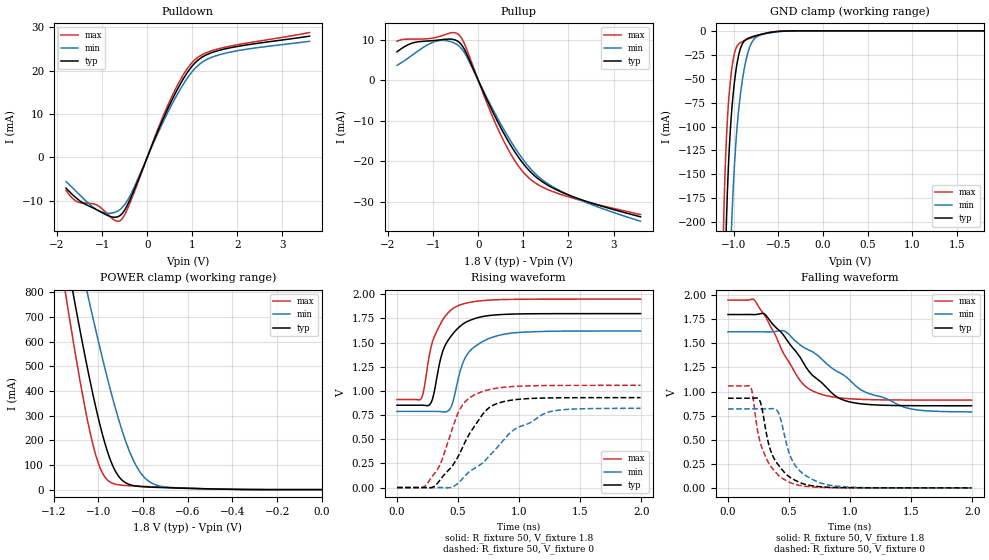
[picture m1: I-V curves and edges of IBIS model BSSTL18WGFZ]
[IBIS Ver] 3.2
[File Name] sprm450.ibs
[File Rev] 1.0
[Date] April 15, 2005
[Source] File Originated at Texas Instruments
[Disclaimer] Please be aware that in the absence of a written agreement
| Texas Instruments(TI) assumes no liability for:
| (1) The accuracy of the IBIS models provided to your company
| (2) The proper functioning of these Models in your design
| or for any resulting applications;or
| (3) Infringement of patents,copyrights, or intellectual
| property rights resulting from your use of these models.
| TI provides IBIS Models as a service to our customers and
| therefore reserves the right to limit distribution of the
| Models.
[Copyright] Property of Texas Instruments Incorporated.
| Unauthorized reproduction and/or distribution is strictly
| prohibited.
| This product is protected under copyright law and trade
| secret law as an unpublished work.
| Created 1999,(C) Copyright 1999-2000,
| Texas Instruments Incorporated., All Rights Reserved.
| These commodities are under the U.S.
| Government distribution license control.As such,they are not
| to be re-exported without the prior approval of the U.S.
| Department of Commerce.
[Notes] DDR Interface for DaVinci only
[Component] TL18WGFZ
[Manufacturer] Texas Instruments
[Package]
|Variable Typ Min Max
R_pkg 2.212e-01 1.101e-01 3.279e-01
L_pkg 4.011e-09 2.375e-09 5.798e-09
C_pkg 6.351e-13 3.910e-13 9.306e-13
[Pin] signal_name model_name
U1 DDR_D_BIT0 BSSTL18WGFZ
U2 DDR_D_BIT1 BSSTL18WGFZ
T5A VDDS1 POWER
W19A VSS GND
V1 DDR_D_BIT2 BSSTL18WGFZ
V2 DDR_D_BIT3 BSSTL18WGFZ
T4 DDR_DQM0 BSSTL18WGFZ
U4 DDR_DQS0 BSSTL18WGFZ
T5B VDDS1 POWER
W19B VSS GND
M12A VDD POWER
W2 DDR_D_BIT4 BSSTL18WGFZ
U3 DDR_D_BIT5 BSSTL18WGFZ
V3 DDR_D_BIT6 BSSTL18WGFZ
W3 DDR_D_BIT7 BSSTL18WGFZ
T5C VDDS1 POWER
W19C VSS GND
V4 DDR_D_BIT8 BSSTL18WGFZ
W4 DDR_D_BIT9 BSSTL18WGFZ
U5 DDR_D_BIT10 BSSTL18WGFZ
V5 DDR_D_BIT11 BSSTL18WGFZ
T5D VDDS1 POWER
W19D VSS GND
U6 DDR_DQS1 BSSTL18WGFZ
T6 DDR_DQM1 BSSTL18WGFZ
W5 DDR_D_BIT12 BSSTL18WGFZ
V6 DDR_D_BIT13 BSSTL18WGFZ
M12B VDD POWER
W19E VSS GND
T5E VDDS1 POWER
W6 DDR_D_BIT14 BSSTL18WGFZ
V7 DDR_D_BIT15 BSSTL18WGFZ
T7 DDR_CAS_N BSSTL18WGFZ
U7 DDR_RAS_N BSSTL18WGFZ
T8 DDR_WE_N BSSTL18WGFZ
W19F VSS GND
T5F VDDS1 POWER
T9 DDR_CS_N BSSTL18WGFZ
V8 DDR_CKE BSSTL18WGFZ
W19G VSS GND
W7 DDR_CLK0 BSSTL18WGFZ
W8 DDR_CLK0_N BSSTL18WGFZ
T5G VDDS1 POWER
W19H VSS GND
M12C VDD POWER
T10 DDR_VDDDLL NC
T11 DDR_VSSDLL NC
R8 DDR_AMUXDLL NC
U9 DDR_BS_BIT2 BSSTL18WGFZ
V9 DDR_BS_BIT1 BSSTL18WGFZ
U8 DDR_BS_BIT0 BSSTL18WGFZ
W19I VSS GND
T5H VDDS1 POWER
W9 DDR_A_BIT12 BSSTL18WGFZ
W10 DDR_A_BIT11 BSSTL18WGFZ
U10 DDR_A_BIT10 BSSTL18WGFZ
U11 DDR_A_BIT9 BSSTL18WGFZ
V10 DDR_A_BIT8 BSSTL18WGFZ
T12 DDR_PADREFN NC
T13 DDR_PADREFP NC
W19J VSS GND
T5I VDDS1 POWER
V11 DDR_A_BIT7 BSSTL18WGFZ
W11 DDR_A_BIT6 BSSTL18WGFZ
W12 DDR_A_BIT5 BSSTL18WGFZ
V12 DDR_A_BIT4 BSSTL18WGFZ
U12 DDR_A_BIT3 BSSTL18WGFZ
M12D VDD POWER
W19K VSS GND
T5J VDDS1 POWER
V13 DDR_A_BIT2 BSSTL18WGFZ
U13 DDR_A_BIT1 BSSTL18WGFZ
W13 DDR_A_BIT0 BSSTL18WGFZ
W14 DDR_D_BIT16 BSSTL18WGFZ
V14 DDR_D_BIT17 BSSTL18WGFZ
W19L VSS GND
T5K VDDS1 POWER
W15 DDR_D_BIT18 BSSTL18WGFZ
V15 DDR_D_BIT19 BSSTL18WGFZ
T14 DDR_DQM2 BSSTL18WGFZ
U14 DDR_DQS2 BSSTL18WGFZ
W19M VSS GND
T5L VDDS1 POWER
U15 DDR_D_BIT20 BSSTL18WGFZ
W16 DDR_D_BIT21 BSSTL18WGFZ
V16 DDR_D_BIT22 BSSTL18WGFZ
T17 DDR_D_BIT23 BSSTL18WGFZ
M12E VDD POWER
W19N VSS GND
T5M VDDS1 POWER
V17 DDR_D_BIT24 BSSTL18WGFZ
U17 DDR_D_BIT25 BSSTL18WGFZ
U18 DDR_D_BIT26 BSSTL18WGFZ
W17 DDR_D_BIT27 BSSTL18WGFZ
W19P VSS GND
T5N VDDS1 POWER
U16 DDR_DQS3 BSSTL18WGFZ
T16 DDR_DQM3 BSSTL18WGFZ
V18 DDR_D_BIT28 BSSTL18WGFZ
W18 DDR_D_BIT29 BSSTL18WGFZ
W19Q VSS GND
T15 VREFSSTL NC
T5P VDDS1 POWER
V19 DDR_D_BIT30 BSSTL18WGFZ
U19 DDR_D_BIT31 BSSTL18WGFZ
[Package Model] ddr
[Define Package Model] ddr
[Manufacturer] Texas Instruments Inc.
[OEM] Texas Instruments Inc.
[Description] Model for ddr generated by PACED 4.51F
[Number of Pins] 105
[Pin Numbers]
U1
U2
T5A
W19A
V1
V2
T4
U4
T5B
W19B
M12A
W2
U3
V3
W3
T5C
W19C
V4
W4
U5
V5
T5D
W19D
U6
T6
W5
V6
M12B
W19E
T5E
W6
V7
T7
U7
T8
W19F
T5F
T9
V8
W19G
W7
W8
T5G
W19H
M12C
T10
T11
R8
U9
V9
U8
W19I
T5H
W9
W10
U10
U11
V10
T12
T13
W19J
T5I
V11
W11
W12
V12
U12
M12D
W19K
T5J
V13
U13
W13
W14
V14
W19L
T5K
W15
V15
T14
U14
W19M
T5L
U15
W16
V16
T17
M12E
W19N
T5M
V17
U17
U18
W17
W19P
T5N
U16
T16
V18
W18
W19Q
T15
T5P
V19
U19
[Model Data]
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[End Model Data]
[End Package Model]
| Models and submodels in the file (1): BSSTL18WGFZ (I/O)
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|[Manufacturer] Texas Instruments.
|[Package]
| variable typ min max
|R_pkg 0.000 0.000 0.000
|L_pkg 0.000H 0.000H 0.000H
|C_pkg 0.000F 0.000F 0.000F
|[Pin] signal_name model_name R_pin L_pin C_pin
|PAD PAD BSSTL18WGFZ NA NA NA
|VDDS VDDS POWER NA NA NA
|VSSS VSSS GND NA NA NA
[Model] BSSTL18WGFZ
Model_type I/O
Polarity Non-Inverting
Enable Active-Low
Vinl = 0.6500V
Vinh = 1.1500V
Vmeas = 0.9000V
Cref = 5.0000pF
Rref = 50.0000
Vref = 0.9000V
| typ min max
|C_comp   1.0539pF   1.0159pF   1.1018pF
|  ADDED 80FF TO C_comp FOR DRIVER TO PAD CAP.
C_comp   1.1339pF   1.0959pF   1.1818pF
[Model Spec]
Vinh 1.1500V 1.0600V 1.2250V
Vinl 0.6500V 0.5600V 0.7250V
[Temperature Range] 25.0000 125.000 -40.0000
[Voltage Range] 1.8000V 1.6200V 1.9500V
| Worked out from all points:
|   slope of the pulldown table from 0 to 0.27 V, typ, clamps not added: 39.3 ohm
|   slope of the pullup table from 0 to 0.27 V, typ, clamps not added: 40.9 ohm
|   GND clamp passes 1 mA (typ) near -0.54 V on its own axis
|   POWER clamp passes 1 mA (typ) near -0.39 V on its own axis
|   rising waveform, R_fixture 50, V_fixture 1.8: 20-80 % time 158ps typ, 161ps min, 144ps max; typ from 0.852 V to 1.8 V
|   falling waveform, R_fixture 50, V_fixture 1.8: 20-80 % time 368ps typ, 595ps min, 266ps max; typ from 1.8 V to 0.852 V
|   rising waveform, R_fixture 50, V_fixture 0: 20-80 % time 267ps typ, 472ps min, 190ps max; typ from 0 V to 0.931 V
|   falling waveform, R_fixture 50, V_fixture 0: 20-80 % time 155ps typ, 156ps min, 143ps max; typ from 0.931 V to 0 V
| (VDD range) 1.100V 0.990V 1.210V
| (Process strength) nominal weak strong
[Pulldown]
|   voltage   I(typ)   I(min)   I(max)
-1.8V     -7.063mA   -5.545mA   -7.599mA
-1.56V    -9.46mA    -7.968mA   -10.15mA
-1.06V    -12.38mA   -12.37mA   -11.29mA
-750mV    -13.76mA   -12.75mA   -14.27mA
-590mV    -13.27mA   -11.88mA   -14.48mA
-360mV    -9.197mA   -8.43mA    -9.903mA
490mV     11.96mA    11.05mA    12.76mA
770mV     17.56mA    16.34mA    18.5mA
1.02V     21.33mA    20.04mA    22.11mA
1.3V      23.57mA    22.44mA    24.06mA
1.7V      24.94mA    23.93mA    25.32mA
3.6V      27.94mA    26.74mA    28.76mA
[GND Clamp]
|   voltage   I(typ)   I(min)   I(max)
-1.8V     -8.153A    -6.587A    -9.945A
-1.12V    -358.5mA   -589mA     -230.2mA
-1.11V    -308.6mA   -534.6mA   -189.8mA
-1.09V    -226.9mA   -435.3mA   -130.7mA
-1.08V    -194.4mA   -390.7mA   -109.4mA
-1.06V    -143.6mA   -311.9mA   -77.56mA
-1.02V    -80.71mA   -195.1mA   -38.47mA
-980mV    -44.92mA   -123.1mA   -19.68mA
-920mV    -17.16mA   -62.89mA   -12.05mA
-820mV    -7.057mA   -16.65mA   -7.987mA
-660mV    -2.917mA   -3.299mA   -2.914mA
1.8V      2.457nA    21.26uA    1.777nA
[Pullup]
|   voltage   I(typ)   I(min)   I(max)
-1.8V     7.006mA    3.659mA    9.604mA
-1.47V    9.129mA    6.125mA    10.14mA
-1V       9.771mA    9.39mA     10.41mA
-480mV    9.77mA     8.861mA    11.58mA
-300mV    7.487mA    6.694mA    8.85mA
210mV     -5.185mA   -4.718mA   -6.092mA
530mV     -12.33mA   -11.4mA    -14.18mA
810mV     -17.63mA   -16.58mA   -19.82mA
1.08V     -21.66mA   -20.78mA   -23.65mA
1.4V      -24.89mA   -24.38mA   -26.22mA
1.84V     -27.57mA   -27.42mA   -28.22mA
3.6V      -33.7mA    -34.81mA   -33.13mA
[POWER Clamp]
|   voltage   I(typ)   I(min)   I(max)
-1.8V     4.591A     4.236A     4.963A
-1.15V    978.1mA    1.219A     809.4mA
-1.14V    927.3mA    1.176A     752.2mA
-1.11V    777.6mA    1.047A     585mA
-1.05V    494.5mA    797.1mA    284.6mA
-1V       287mA      599.3mA    105.2mA
-940mV    104.8mA    381.8mA    26.8mA
-900mV    43.34mA    255.7mA    18.24mA
-840mV    15.65mA    111.9mA    14.67mA
-800mV    11.58mA    54.84mA    13.09mA
-750mV    9.389mA    21.52mA    11.23mA
0V        2.457nA    21.62nA    3.9nA
[Ramp]
|parameter   typ   min   max
dV/dt_r   0.5584/0.2658n   0.4921/0.4699n   0.6349/0.1906n
dV/dt_f   0.5687/0.3681n   0.4992/0.5988n   0.6232/0.2659n
R_load = 50ohms
[Rising Waveform]
R_fixture = 50
V_fixture = 1.8
V_fixture_min = 1.62
V_fixture_max = 1.95
|   time   V(typ)   V(min)   V(max)
0s        852.1mV    787.9mV    911.3mV
195ps     852.5mV    787.9mV    915.9mV
265ps     854.4mV    787.8mV    1.369V
300ps     960.9mV    788mV      1.544V
370ps     1.391V     784.1mV    1.725V
430ps     1.545V     807mV      1.823V
500ps     1.649V     1.117V     1.882V
595ps     1.729V     1.41V      1.916V
815ps     1.787V     1.568V     1.943V
1.995ns   1.8V       1.62V      1.95V
[Falling Waveform]
R_fixture = 50
V_fixture = 1.8
V_fixture_min = 1.62
V_fixture_max = 1.95
|   time   V(typ)   V(min)   V(max)
0s        1.8V       1.62V      1.95V
215ps     1.799V     1.62V      1.952V
300ps     1.804V     1.62V      1.793V
460ps     1.576V     1.63V      1.385V
590ps     1.358V     1.485V     1.115V
740ps     1.12V      1.37V      981.7mV
965ps     903.1mV    1.155V     928.1mV
1.11ns    870.3mV    1.003V     918mV
1.43ns    854.3mV    844.3mV    912.3mV
1.995ns   852.3mV    789mV      911.4mV
[Rising Waveform]
R_fixture = 50
V_fixture = 0
|   time   V(typ)   V(min)   V(max)
0s        2.706uV    19.8uV     1.231uV
245ps     -1.367mV   30.45uV    36.13mV
360ps     91.2mV     495uV      259.2mV
510ps     344.4mV    56.44mV    798.6mV
655ps     672.4mV    213.2mV    972.1mV
730ps     799.9mV    291mV      1.006V
815ps     867.2mV    406.9mV    1.028V
950ps     906.5mV    591.4mV    1.046V
1.225ns   927.1mV    774.5mV    1.056V
1.995ns   930.6mV    820mV      1.058V
[Falling Waveform]
R_fixture = 50
V_fixture = 0
|   time   V(typ)   V(min)   V(max)
0s        930.8mV    820.3mV    1.058V
185ps     930.6mV    820.3mV    1.048V
200ps     930.3mV    820.3mV    981mV
260ps     907mV      820.4mV    487.8mV
340ps     423.5mV    821.1mV    243.3mV
410ps     241.2mV    788.6mV    133.8mV
515ps     103.6mV    314.7mV    52.05mV
625ps     38.88mV    137.6mV    17.73mV
840ps     5.3mV      26.45mV    2.166mV
1.995ns   110.9uV    134.2uV    93.86uV
